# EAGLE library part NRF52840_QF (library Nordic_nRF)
nRF52840 Features Advanced Single chip 2.4 GHz multi-protocol SoC 32-bit ARM Cortex-M4F Processor 1.7v to 5.5v operation 1MB flash + 256kB RAM Bluetooth 5 support for long range and high throughput 802.15.4 radio support On-chip NFC PPI –Programmable Peripheral Interconnect Automated power management system with automatic power management of each peripheral Configurable I/O mapping for analog and digital I/O 48 x GPIO 1 x QSPI 4 x Master/Slave SPI 2 x Two-wire interface (I²C) I²S interface 2 x UART 4 x PWM USB 2.0 controller ARM TrustZone CryptoCell-310 Cryptographic and security module AES 128-bit ECB/CCM/AAR hardware accelerator Digital microphone interface (PDM) Quadrature decoder 12-bit ADC Low power comparator On-chip 50Ω balun On-air compatible with nRF52, nRF51 and nRF24 Series Applications Advanced high performance wearables Wearables for secure payments Virtual Reality/Augmented Reality systems Smart Home sensor networks Smart city sensor networks High performance HID controllers Internet of Things (IoT) sensor networks Smart door locks Smart lighting networks Connected white goods
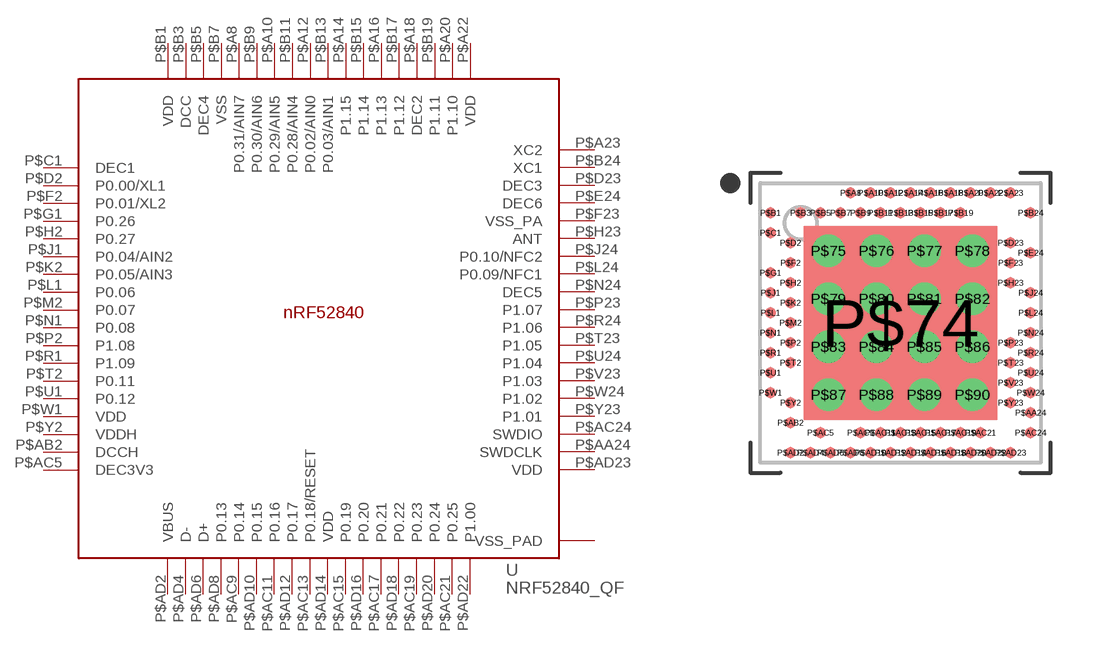
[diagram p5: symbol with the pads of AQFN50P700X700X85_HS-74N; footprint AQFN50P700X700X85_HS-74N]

Designator prefix -

## NRF52840_QF  [AQFN50P700X700X85_HS-74N]
P$74  VSS_PAD
P$75  VSS_PAD
P$76  VSS_PAD
P$77  VSS_PAD
P$78  VSS_PAD
P$79  VSS_PAD
P$80  VSS_PAD
P$81  VSS_PAD
P$82  VSS_PAD
P$83  VSS_PAD
P$84  VSS_PAD
P$85  VSS_PAD
P$86  VSS_PAD
P$87  VSS_PAD
P$88  VSS_PAD
P$89  VSS_PAD
P$90  VSS_PAD
P$A8  P0.31/AIN7
P$A10  P0.29/AIN5
P$A12  P0.02/AIN0
P$A14  P1.15
P$A16  P1.13
P$A18  DEC2
P$A20  P1.10
P$A22  VDD  pwr
P$A23  XC2  out
P$AA24  SWDCLK  in
P$AB2  DCCH
P$AC5  DEC3V3
P$AC9  P0.14
P$AC11  P0.16
P$AC13  P0.18/RESET
P$AC15  P0.19
P$AC17  P0.21
P$AC19  P0.23
P$AC21  P0.25
P$AC24  SWDIO
P$AD2  VBUS  pwr
P$AD4  D-
P$AD6  D+
P$AD8  P0.13
P$AD10  P0.15
P$AD12  P0.17
P$AD14  VDD  pwr
P$AD16  P0.20
P$AD18  P0.22
P$AD20  P0.24
P$AD22  P1.00
P$AD23  VDD  pwr
P$B1  VDD  pwr
P$B3  DCC  out
P$B5  DEC4  pwr
P$B7  VSS  pwr
P$B9  P0.30/AIN6
P$B11  P0.28/AIN4
P$B13  P0.03/AIN1
P$B15  P1.14
P$B17  P1.12
P$B19  P1.11
P$B24  XC1  in
P$C1  DEC1  pwr
P$D2  P0.00/XL1
P$D23  DEC3
P$E24  DEC6
P$F2  P0.01/XL2
P$F23  VSS_PA
P$G1  P0.26
P$H2  P0.27
P$H23  ANT
P$J1  P0.04/AIN2
P$J24  P0.10/NFC2
P$K2  P0.05/AIN3
P$L1  P0.06
P$L24  P0.09/NFC1
P$M2  P0.07
P$N1  P0.08
P$N24  DEC5
P$P2  P1.08
P$P23  P1.07
P$R1  P1.09
P$R24  P1.06
P$T2  P0.11
P$T23  P1.05
P$U1  P0.12
P$U24  P1.04
P$V23  P1.03
P$W1  VDD  pwr
P$W24  P1.02
P$Y2  VDDH  pwr
P$Y23  P1.01

## Footprint AQFN50P700X700X85_HS-74N (pad centres in mm)
smd 4.85 x 4.85: P$74 0,0
drill 0.3 pad 0.6: P$75 -1.8,1.8; P$76 -0.6,1.8; P$77 0.6,1.8; P$78 1.8,1.8; P$79 -1.8,0.6; P$80 -0.6,0.6; P$81 0.6,0.6; P$82 1.8,0.6; P$83 -1.8,-0.6; P$84 -0.6,-0.6; P$85 0.6,-0.6; P$86 1.8,-0.6; P$87 -1.8,-1.8; P$88 -0.6,-1.8; P$89 0.6,-1.8; P$90 1.8,-1.8
smd 0.275 x 0.275: P$A8 -1.25,3.25; P$A10 -0.75,3.25; P$A12 -0.25,3.25; P$A14 0.25,3.25; P$A16 0.75,3.25; P$A18 1.25,3.25; P$A20 1.75,3.25; P$A22 2.25,3.25; P$A23 2.75,3.25; P$AA24 3.25,-2.25; P$AB2 -2.75,-2.5; P$AC5 -2,-2.75; P$AC9 -1,-2.75; P$AC11 -0.5,-2.75; P$AC13 0,-2.75; P$AC15 0.5,-2.75; P$AC17 1,-2.75; P$AC19 1.5,-2.75; P$AC21 2,-2.75; P$AC24 3.25,-2.75; P$AD2 -2.75,-3.25; P$AD4 -2.25,-3.25; P$AD6 -1.75,-3.25; P$AD8 -1.25,-3.25; P$AD10 -0.75,-3.25; P$AD12 -0.25,-3.25; P$AD14 0.25,-3.25; P$AD16 0.75,-3.25; P$AD18 1.25,-3.25; P$AD20 1.75,-3.25; P$AD22 2.25,-3.25; P$AD23 2.75,-3.25; P$B1 -3.25,2.75; P$B3 -2.5,2.75; P$B5 -2,2.75; P$B7 -1.5,2.75; P$B9 -1,2.75; P$B11 -0.5,2.75; P$B13 0,2.75; P$B15 0.5,2.75; P$B17 1,2.75; P$B19 1.5,2.75; P$B24 3.25,2.75; P$C1 -3.25,2.25; P$D2 -2.75,2; P$D23 2.75,2; P$E24 3.25,1.75; P$F2 -2.75,1.5; P$F23 2.75,1.5; P$G1 -3.25,1.25; P$H2 -2.75,1; P$H23 2.75,1; P$J1 -3.25,0.75; P$J24 3.25,0.75; P$K2 -2.75,0.5; P$L1 -3.25,0.25; P$L24 3.25,0.25; P$M2 -2.75,0; P$N1 -3.25,-0.25; P$N24 3.25,-0.25; P$P2 -2.75,-0.5; P$P23 2.75,-0.5; P$R1 -3.25,-0.75; P$R24 3.25,-0.75; P$T2 -2.75,-1; P$T23 2.75,-1; P$U1 -3.25,-1.25; P$U24 3.25,-1.25; P$V23 2.75,-1.5; P$W1 -3.25,-1.75; P$W24 3.25,-1.75; P$Y2 -2.75,-2; P$Y23 2.75,-2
